| IBIS file stm32u575_585_ufqfpn48.ibs
[IBIS ver] 4.2
[File name] stm32u575_585_ufqfpn48.ibs
[File Rev] 1.0
[Date]   06-08-2021
[Source] Data Created at STMicroelectronics
[Notes]  File originated from ELDO simulations.
[Disclaimer]  This information is for modeling purpose only and is
   not guaranted. The information is subject to change without
   notice.
[Copyright] Copyright 2021 STMicroelectronics Inc.
|   Component stm32u575_585_ufqfpn48
[Component] stm32u575_585_ufqfpn48
[Manufacturer] STMicroelectronics
[Package]
| variable   typ   min   max
R_pkg   0   NA   NA
L_pkg   0   NA   NA
C_pkg   0   NA   NA
[Pin]   signal_name   model_name   R_pin   L_pin   C_pin   | Comment
1 VBAT POWER
2 PC13 io8_100m_ft_v33
3 PC14-OSC32_IN io8_100m_ft
4 PC15-OSC32_OUT io8_100m_ft
5 PH0-OSC_IN io8_100m_ft
6 PH1-OSC_OUT io8_100m_ft
7 NRST nc
8 VSSA GND
9 VDDA POWER
10 PA0 io8_100m_hslv_tamp_ft
11 PA1 io8_100m_hslv_tamp_ft
12 PA2 io8_100m_hslv_ft
13 PA3 io8_166m_hslv_ft
14 PA4 io8_100m_hslv_ft
15 PA5 io8_100m_ft
16 PA6 io8_100m_hslv_ft
17 PA7 io8_100m_hslv_ft
18 PB0 io8_100m_hslv_ft
19 PB1 io8_100m_hslv_ft
20 PB2 io8_100m_hslv_tamp_ft
21 PB10 io8_166m_hslv_i2c_ft
22 VCAP POWER
23 VSS GND
24 VDD POWER
25 PB12 io8_166m_hslv_ft
26 PB13 io8_100m_i2c_ft
27 PB14 io8_100m_i2c_ft
28 PB15 nc
29 PA8 io8_166m_hslv_ft
30 PA9 io8_100m_usb_vbus_ft
31 PA10 io8_100m_usb_id
32 PA11 io8_usb_ft
33 PA12 io8_usb_ft
34 PA13 io8_100m_ft
35 VSS GND
36 VDD POWER
37 PA14 io8_100m_ft
38 PA15 nc
39 PB3 io8_100m_i2c_ft
40 PB4 io8_100m_i2c_ft
41 PB5 io8_166m_hslv_ft
42 PB6 io8_100m_i2c_ft
43 PB7 io8_166m_hslv_i2c_ft
44 PH3-BOOT0 io8_100m_ft
45 PB8 io8_100m_i2c_ft
46 PB9 io8_100m_i2c_ft
47 VSS GND
48 VDD POWER
[Model Selector] io8_100m_ft
io8_100m_ft_hs_1v2  "IO8_FT 100MHz high speed @ 1.2V"
io8_100m_ft_hs_pu_1v2  "IO8_FT 100MHz high speed @ 1.2V pullup"
io8_100m_ft_hs_pd_1v2  "IO8_FT 100MHz high speed @ 1.2V pulldown"
io8_100m_ft_fs_1v2  "IO8_FT 100MHz fast speed @ 1.2V"
io8_100m_ft_fs_pu_1v2  "IO8_FT 100MHz fast speed @ 1.2V pullup"
io8_100m_ft_fs_pd_1v2  "IO8_FT 100MHz fast speed @ 1.2V pulldown"
io8_100m_ft_ms_1v2  "IO8_FT 100MHz med speed @ 1.2V"
io8_100m_ft_ms_pu_1v2  "IO8_FT 100MHz med speed @ 1.2V pullup"
io8_100m_ft_ms_pd_1v2  "IO8_FT 100MHz med speed @ 1.2V pulldown"
io8_100m_ft_ls_1v2  "IO8_FT 100MHz low speed @ 1.2V"
io8_100m_ft_ls_pu_1v2  "IO8_FT 100MHz low speed @ 1.2V pullup"
io8_100m_ft_ls_pd_1v2  "IO8_FT 100MHz low speed @ 1.2V pulldown"
io8_100m_ft_hs_1v8  "IO8_FT 100MHz high speed @ 1.8V"
io8_100m_ft_hs_pu_1v8  "IO8_FT 100MHz high speed @ 1.8V pullup"
io8_100m_ft_hs_pd_1v8  "IO8_FT 100MHz high speed @ 1.8V pulldown"
io8_100m_ft_fs_1v8  "IO8_FT 100MHz fast speed @ 1.8V"
io8_100m_ft_fs_pu_1v8  "IO8_FT 100MHz fast speed @ 1.8V pullup"
io8_100m_ft_fs_pd_1v8  "IO8_FT 100MHz fast speed @ 1.8V pulldown"
io8_100m_ft_ms_1v8  "IO8_FT 100MHz med speed @ 1.8V"
io8_100m_ft_ms_pu_1v8  "IO8_FT 100MHz med speed @ 1.8V pullup"
io8_100m_ft_ms_pd_1v8  "IO8_FT 100MHz med speed @ 1.8V pulldown"
io8_100m_ft_ls_1v8  "IO8_FT 100MHz low speed @ 1.8V"
io8_100m_ft_ls_pu_1v8  "IO8_FT 100MHz low speed @ 1.8V pullup"
io8_100m_ft_ls_pd_1v8  "IO8_FT 100MHz low speed @ 1.8V pulldown"
io8_100m_ft_hs_3v3  "IO8_FT 100MHz high speed @ 3.3V"
io8_100m_ft_hs_pu_3v3  "IO8_FT 100MHz high speed @ 3.3V pullup"
io8_100m_ft_hs_pd_3v3  "IO8_FT 100MHz high speed @ 3.3V pulldown"
io8_100m_ft_fs_3v3  "IO8_FT 100MHz fast speed @ 3.3V"
io8_100m_ft_fs_pu_3v3  "IO8_FT 100MHz fast speed @ 3.3V pullup"
io8_100m_ft_fs_pd_3v3  "IO8_FT 100MHz fast speed @ 3.3V pulldown"
io8_100m_ft_ms_3v3  "IO8_FT 100MHz med speed @ 3.3V"
io8_100m_ft_ms_pu_3v3  "IO8_FT 100MHz med speed @ 3.3V pullup"
io8_100m_ft_ms_pd_3v3  "IO8_FT 100MHz med speed @ 3.3V pulldown"
io8_100m_ft_ls_3v3  "IO8_FT 100MHz low speed @ 3.3V"
io8_100m_ft_ls_pu_3v3  "IO8_FT 100MHz low speed @ 3.3V pullup"
io8_100m_ft_ls_pd_3v3  "IO8_FT 100MHz low speed @ 3.3V pulldown"
[Model Selector] io8_100m_hslv_ft
io8_100m_ft_hs_1v2  "IO8_FT 100MHz high speed @ 1.2V"
io8_100m_ft_hs_pu_1v2  "IO8_FT 100MHz high speed @ 1.2V pullup"
io8_100m_ft_hs_pd_1v2  "IO8_FT 100MHz high speed @ 1.2V pulldown"
io8_100m_ft_fs_1v2  "IO8_FT 100MHz fast speed @ 1.2V"
io8_100m_ft_fs_pu_1v2  "IO8_FT 100MHz fast speed @ 1.2V pullup"
io8_100m_ft_fs_pd_1v2  "IO8_FT 100MHz fast speed @ 1.2V pulldown"
io8_100m_ft_ms_1v2  "IO8_FT 100MHz med speed @ 1.2V"
io8_100m_ft_ms_pu_1v2  "IO8_FT 100MHz med speed @ 1.2V pullup"
io8_100m_ft_ms_pd_1v2  "IO8_FT 100MHz med speed @ 1.2V pulldown"
io8_100m_ft_ls_1v2  "IO8_FT 100MHz low speed @ 1.2V"
io8_100m_ft_ls_pu_1v2  "IO8_FT 100MHz low speed @ 1.2V pullup"
io8_100m_ft_ls_pd_1v2  "IO8_FT 100MHz low speed @ 1.2V pulldown"
io8_100m_ft_hs_1v8  "IO8_FT 100MHz high speed @ 1.8V"
io8_100m_ft_hs_pu_1v8  "IO8_FT 100MHz high speed @ 1.8V pullup"
io8_100m_ft_hs_pd_1v8  "IO8_FT 100MHz high speed @ 1.8V pulldown"
io8_100m_ft_fs_1v8  "IO8_FT 100MHz fast speed @ 1.8V"
io8_100m_ft_fs_pu_1v8  "IO8_FT 100MHz fast speed @ 1.8V pullup"
io8_100m_ft_fs_pd_1v8  "IO8_FT 100MHz fast speed @ 1.8V pulldown"
io8_100m_ft_ms_1v8  "IO8_FT 100MHz med speed @ 1.8V"
io8_100m_ft_ms_pu_1v8  "IO8_FT 100MHz med speed @ 1.8V pullup"
io8_100m_ft_ms_pd_1v8  "IO8_FT 100MHz med speed @ 1.8V pulldown"
io8_100m_ft_ls_1v8  "IO8_FT 100MHz low speed @ 1.8V"
io8_100m_ft_ls_pu_1v8  "IO8_FT 100MHz low speed @ 1.8V pullup"
io8_100m_ft_ls_pd_1v8  "IO8_FT 100MHz low speed @ 1.8V pulldown"
io8_100m_ft_hs_3v3  "IO8_FT 100MHz high speed @ 3.3V"
io8_100m_ft_hs_pu_3v3  "IO8_FT 100MHz high speed @ 3.3V pullup"
io8_100m_ft_hs_pd_3v3  "IO8_FT 100MHz high speed @ 3.3V pulldown"
io8_100m_ft_fs_3v3  "IO8_FT 100MHz fast speed @ 3.3V"
io8_100m_ft_fs_pu_3v3  "IO8_FT 100MHz fast speed @ 3.3V pullup"
io8_100m_ft_fs_pd_3v3  "IO8_FT 100MHz fast speed @ 3.3V pulldown"
io8_100m_ft_ms_3v3  "IO8_FT 100MHz med speed @ 3.3V"
io8_100m_ft_ms_pu_3v3  "IO8_FT 100MHz med speed @ 3.3V pullup"
io8_100m_ft_ms_pd_3v3  "IO8_FT 100MHz med speed @ 3.3V pulldown"
io8_100m_ft_ls_3v3  "IO8_FT 100MHz low speed @ 3.3V"
io8_100m_ft_ls_pu_3v3  "IO8_FT 100MHz low speed @ 3.3V pullup"
io8_100m_ft_ls_pd_3v3  "IO8_FT 100MHz low speed @ 3.3V pulldown"
io8_100m_hslv_ft_hs_1v2  "IO8_FT 100MHz HSLV high speed @ 1.2V"
io8_100m_hslv_ft_hs_pu_1v2  "IO8_FT 100MHz HSLV high speed @ 1.2V pullup"
io8_100m_hslv_ft_hs_pd_1v2  "IO8_FT 100MHz HSLV high speed @ 1.2V pulldown"
io8_100m_hslv_ft_fs_1v2  "IO8_FT 100MHz HSLV fast speed @ 1.2V"
io8_100m_hslv_ft_fs_pu_1v2  "IO8_FT 100MHz HSLV fast speed @ 1.2V pullup"
io8_100m_hslv_ft_fs_pd_1v2  "IO8_FT 100MHz HSLV fast speed @ 1.2V pulldown"
io8_100m_hslv_ft_ms_1v2  "IO8_FT 100MHz HSLV med speed @ 1.2V"
io8_100m_hslv_ft_ms_pu_1v2  "IO8_FT 100MHz HSLV med speed @ 1.2V pullup"
io8_100m_hslv_ft_ms_pd_1v2  "IO8_FT 100MHz HSLV med speed @ 1.2V pulldown"
io8_100m_hslv_ft_ls_1v2  "IO8_FT 100MHz HSLV low speed @ 1.2V"
io8_100m_hslv_ft_ls_pu_1v2  "IO8_FT 100MHz HSLV low speed @ 1.2V pullup"
io8_100m_hslv_ft_ls_pd_1v2  "IO8_FT 100MHz HSLV low speed @ 1.2V pulldown"
io8_100m_hslv_ft_hs_1v8  "IO8_FT 100MHz HSLV high speed @ 1.8V"
io8_100m_hslv_ft_hs_pu_1v8  "IO8_FT 100MHz HSLV high speed @ 1.8V pullup"
io8_100m_hslv_ft_hs_pd_1v8  "IO8_FT 100MHz HSLV high speed @ 1.8V pulldown"
io8_100m_hslv_ft_fs_1v8  "IO8_FT 100MHz HSLV fast speed @ 1.8V"
io8_100m_hslv_ft_fs_pu_1v8  "IO8_FT 100MHz HSLV fast speed @ 1.8V pullup"
io8_100m_hslv_ft_fs_pd_1v8  "IO8_FT 100MHz HSLV fast speed @ 1.8V pulldown"
io8_100m_hslv_ft_ms_1v8  "IO8_FT 100MHz HSLV med speed @ 1.8V"
io8_100m_hslv_ft_ms_pu_1v8  "IO8_FT 100MHz HSLV med speed @ 1.8V pullup"
io8_100m_hslv_ft_ms_pd_1v8  "IO8_FT 100MHz HSLV med speed @ 1.8V pulldown"
io8_100m_hslv_ft_ls_1v8  "IO8_FT 100MHz HSLV low speed @ 1.8V"
io8_100m_hslv_ft_ls_pu_1v8  "IO8_FT 100MHz HSLV low speed @ 1.8V pullup"
io8_100m_hslv_ft_ls_pd_1v8  "IO8_FT 100MHz HSLV low speed @ 1.8V pulldown"
io8_100m_hslv_ft_hs_2v5  "IO8_FT 100MHz HSLV high speed @ 2.5V"
io8_100m_hslv_ft_hs_pu_2v5  "IO8_FT 100MHz HSLV high speed @ 2.5V pullup"
io8_100m_hslv_ft_hs_pd_2v5  "IO8_FT 100MHz HSLV high speed @ 2.5V pulldown"
io8_100m_hslv_ft_fs_2v5  "IO8_FT 100MHz HSLV fast speed @ 2.5V"
io8_100m_hslv_ft_fs_pu_2v5  "IO8_FT 100MHz HSLV fast speed @ 2.5V pullup"
io8_100m_hslv_ft_fs_pd_2v5  "IO8_FT 100MHz HSLV fast speed @ 2.5V pulldown"
io8_100m_hslv_ft_ms_2v5  "IO8_FT 100MHz HSLV med speed @ 2.5V"
io8_100m_hslv_ft_ms_pu_2v5  "IO8_FT 100MHz HSLV med speed @ 2.5V pullup"
io8_100m_hslv_ft_ms_pd_2v5  "IO8_FT 100MHz HSLV med speed @ 2.5V pulldown"
io8_100m_hslv_ft_ls_2v5  "IO8_FT 100MHz HSLV low speed @ 2.5V"
io8_100m_hslv_ft_ls_pu_2v5  "IO8_FT 100MHz HSLV low speed @ 2.5V pullup"
io8_100m_hslv_ft_ls_pd_2v5  "IO8_FT 100MHz HSLV low speed @ 2.5V pulldown"
[Model Selector] io8_166m_hslv_ft
io8_166m_ft_hs_1v2  "IO8_FT 166MHz high speed @ 1.2V"
io8_166m_ft_hs_pu_1v2  "IO8_FT 166MHz high speed @ 1.2V pullup"
io8_166m_ft_hs_pd_1v2  "IO8_FT 166MHz high speed @ 1.2V pulldown"
io8_166m_ft_fs_1v2  "IO8_FT 166MHz fast speed @ 1.2V"
io8_166m_ft_fs_pu_1v2  "IO8_FT 166MHz fast speed @ 1.2V pullup"
io8_166m_ft_fs_pd_1v2  "IO8_FT 166MHz fast speed @ 1.2V pulldown"
io8_166m_ft_ms_1v2  "IO8_FT 166MHz med speed @ 1.2V"
io8_166m_ft_ms_pu_1v2  "IO8_FT 166MHz med speed @ 1.2V pullup"
io8_166m_ft_ms_pd_1v2  "IO8_FT 166MHz med speed @ 1.2V pulldown"
io8_166m_ft_ls_1v2  "IO8_FT 166MHz low speed @ 1.2V"
io8_166m_ft_ls_pu_1v2  "IO8_FT 166MHz low speed @ 1.2V pullup"
io8_166m_ft_ls_pd_1v2  "IO8_FT 166MHz low speed @ 1.2V pulldown"
io8_166m_ft_hs_1v8  "IO8_FT 166MHz high speed @ 1.8V"
io8_166m_ft_hs_pu_1v8  "IO8_FT 166MHz high speed @ 1.8V pullup"
io8_166m_ft_hs_pd_1v8  "IO8_FT 166MHz high speed @ 1.8V pulldown"
io8_166m_ft_fs_1v8  "IO8_FT 166MHz fast speed @ 1.8V"
io8_166m_ft_fs_pu_1v8  "IO8_FT 166MHz fast speed @ 1.8V pullup"
io8_166m_ft_fs_pd_1v8  "IO8_FT 166MHz fast speed @ 1.8V pulldown"
io8_166m_ft_ms_1v8  "IO8_FT 166MHz med speed @ 1.8V"
io8_166m_ft_ms_pu_1v8  "IO8_FT 166MHz med speed @ 1.8V pullup"
io8_166m_ft_ms_pd_1v8  "IO8_FT 166MHz med speed @ 1.8V pulldown"
io8_166m_ft_ls_1v8  "IO8_FT 166MHz low speed @ 1.8V"
io8_166m_ft_ls_pu_1v8  "IO8_FT 166MHz low speed @ 1.8V pullup"
io8_166m_ft_ls_pd_1v8  "IO8_FT 166MHz low speed @ 1.8V pulldown"
io8_166m_ft_hs_3v3  "IO8_FT 166MHz high speed @ 3.3V"
io8_166m_ft_hs_pu_3v3  "IO8_FT 166MHz high speed @ 3.3V pullup"
io8_166m_ft_hs_pd_3v3  "IO8_FT 166MHz high speed @ 3.3V pulldown"
io8_166m_ft_fs_3v3  "IO8_FT 166MHz fast speed @ 3.3V"
io8_166m_ft_fs_pu_3v3  "IO8_FT 166MHz fast speed @ 3.3V pullup"
io8_166m_ft_fs_pd_3v3  "IO8_FT 166MHz fast speed @ 3.3V pulldown"
io8_166m_ft_ms_3v3  "IO8_FT 166MHz med speed @ 3.3V"
io8_166m_ft_ms_pu_3v3  "IO8_FT 166MHz med speed @ 3.3V pullup"
io8_166m_ft_ms_pd_3v3  "IO8_FT 166MHz med speed @ 3.3V pulldown"
io8_166m_ft_ls_3v3  "IO8_FT 166MHz low speed @ 3.3V"
io8_166m_ft_ls_pu_3v3  "IO8_FT 166MHz low speed @ 3.3V pullup"
io8_166m_ft_ls_pd_3v3  "IO8_FT 166MHz low speed @ 3.3V pulldown"
io8_166m_hslv_ft_hs_1v2  "IO8_FT 166MHz HSLV high speed @ 1.2V"
io8_166m_hslv_ft_hs_pu_1v2  "IO8_FT 166MHz HSLV high speed @ 1.2V pullup"
io8_166m_hslv_ft_hs_pd_1v2  "IO8_FT 166MHz HSLV high speed @ 1.2V pulldown"
io8_166m_hslv_ft_fs_1v2  "IO8_FT 166MHz HSLV fast speed @ 1.2V"
io8_166m_hslv_ft_fs_pu_1v2  "IO8_FT 166MHz HSLV fast speed @ 1.2V pullup"
io8_166m_hslv_ft_fs_pd_1v2  "IO8_FT 166MHz HSLV fast speed @ 1.2V pulldown"
io8_166m_hslv_ft_ms_1v2  "IO8_FT 166MHz HSLV med speed @ 1.2V"
io8_166m_hslv_ft_ms_pu_1v2  "IO8_FT 166MHz HSLV med speed @ 1.2V pullup"
io8_166m_hslv_ft_ms_pd_1v2  "IO8_FT 166MHz HSLV med speed @ 1.2V pulldown"
io8_166m_hslv_ft_ls_1v2  "IO8_FT 166MHz HSLV low speed @ 1.2V"
io8_166m_hslv_ft_ls_pu_1v2  "IO8_FT 166MHz HSLV low speed @ 1.2V pullup"
io8_166m_hslv_ft_ls_pd_1v2  "IO8_FT 166MHz HSLV low speed @ 1.2V pulldown"
io8_166m_hslv_ft_hs_1v8  "IO8_FT 166MHz HSLV high speed @ 1.8V"
io8_166m_hslv_ft_hs_pu_1v8  "IO8_FT 166MHz HSLV high speed @ 1.8V pullup"
io8_166m_hslv_ft_hs_pd_1v8  "IO8_FT 166MHz HSLV high speed @ 1.8V pulldown"
io8_166m_hslv_ft_fs_1v8  "IO8_FT 166MHz HSLV fast speed @ 1.8V"
io8_166m_hslv_ft_fs_pu_1v8  "IO8_FT 166MHz HSLV fast speed @ 1.8V pullup"
io8_166m_hslv_ft_fs_pd_1v8  "IO8_FT 166MHz HSLV fast speed @ 1.8V pulldown"
io8_166m_hslv_ft_ms_1v8  "IO8_FT 166MHz HSLV med speed @ 1.8V"
io8_166m_hslv_ft_ms_pu_1v8  "IO8_FT 166MHz HSLV med speed @ 1.8V pullup"
io8_166m_hslv_ft_ms_pd_1v8  "IO8_FT 166MHz HSLV med speed @ 1.8V pulldown"
io8_166m_hslv_ft_ls_1v8  "IO8_FT 166MHz HSLV low speed @ 1.8V"
io8_166m_hslv_ft_ls_pu_1v8  "IO8_FT 166MHz HSLV low speed @ 1.8V pullup"
io8_166m_hslv_ft_ls_pd_1v8  "IO8_FT 166MHz HSLV low speed @ 1.8V pulldown"
io8_166m_hslv_ft_hs_2v5  "IO8_FT 166MHz HSLV high speed @ 2.5V"
io8_166m_hslv_ft_hs_pu_2v5  "IO8_FT 166MHz HSLV high speed @ 2.5V pullup"
io8_166m_hslv_ft_hs_pd_2v5  "IO8_FT 166MHz HSLV high speed @ 2.5V pulldown"
io8_166m_hslv_ft_fs_2v5  "IO8_FT 166MHz HSLV fast speed @ 2.5V"
io8_166m_hslv_ft_fs_pu_2v5  "IO8_FT 166MHz HSLV fast speed @ 2.5V pullup"
io8_166m_hslv_ft_fs_pd_2v5  "IO8_FT 166MHz HSLV fast speed @ 2.5V pulldown"
io8_166m_hslv_ft_ms_2v5  "IO8_FT 166MHz HSLV med speed @ 2.5V"
io8_166m_hslv_ft_ms_pu_2v5  "IO8_FT 166MHz HSLV med speed @ 2.5V pullup"
io8_166m_hslv_ft_ms_pd_2v5  "IO8_FT 166MHz HSLV med speed @ 2.5V pulldown"
io8_166m_hslv_ft_ls_2v5  "IO8_FT 166MHz HSLV low speed @ 2.5V"
io8_166m_hslv_ft_ls_pu_2v5  "IO8_FT 166MHz HSLV low speed @ 2.5V pullup"
io8_166m_hslv_ft_ls_pd_2v5  "IO8_FT 166MHz HSLV low speed @ 2.5V pulldown"
[Model Selector] io8_100m_ft_v33
io8_ft_v33_hs_1v2  "IO8_FT_V33 high speed @ 1.2V"
io8_ft_v33_hs_pu_1v2  "IO8_FT_V33 high speed @ 1.2V pullup"
io8_ft_v33_hs_pd_1v2  "IO8_FT_V33 high speed @ 1.2V pulldown"
io8_ft_v33_fs_1v2  "IO8_FT_V33 fast speed @ 1.2V"
io8_ft_v33_fs_pu_1v2  "IO8_FT_V33 fast speed @ 1.2V pullup"
io8_ft_v33_fs_pd_1v2  "IO8_FT_V33 fast speed @ 1.2V pulldown"
io8_ft_v33_ms_1v2  "IO8_FT_V33 med speed @ 1.2V"
io8_ft_v33_ms_pu_1v2  "IO8_FT_V33 med speed @ 1.2V pullup"
io8_ft_v33_ms_pd_1v2  "IO8_FT_V33 med speed @ 1.2V pulldown"
io8_ft_v33_ls_1v2  "IO8_FT_V33 low speed @ 1.2V"
io8_ft_v33_ls_pu_1v2  "IO8_FT_V33 low speed @ 1.2V pullup"
io8_ft_v33_ls_pd_1v2  "IO8_FT_V33 low speed @ 1.2V pulldown"
io8_ft_v33_hs_1v8  "IO8_FT_V33 high speed @ 1.8V"
io8_ft_v33_hs_pu_1v8  "IO8_FT_V33 high speed @ 1.8V pullup"
io8_ft_v33_hs_pd_1v8  "IO8_FT_V33 high speed @ 1.8V pulldown"
io8_ft_v33_fs_1v8  "IO8_FT_V33 fast speed @ 1.8V"
io8_ft_v33_fs_pu_1v8  "IO8_FT_V33 fast speed @ 1.8V pullup"
io8_ft_v33_fs_pd_1v8  "IO8_FT_V33 fast speed @ 1.8V pulldown"
io8_ft_v33_ms_1v8  "IO8_FT_V33 med speed @ 1.8V"
io8_ft_v33_ms_pu_1v8  "IO8_FT_V33 med speed @ 1.8V pullup"
io8_ft_v33_ms_pd_1v8  "IO8_FT_V33 med speed @ 1.8V pulldown"
io8_ft_v33_ls_1v8  "IO8_FT_V33 low speed @ 1.8V"
io8_ft_v33_ls_pu_1v8  "IO8_FT_V33 low speed @ 1.8V pullup"
io8_ft_v33_ls_pd_1v8  "IO8_FT_V33 low speed @ 1.8V pulldown"
io8_ft_v33_hs_3v3  "IO8_FT_V33 high speed @ 3.3V"
io8_ft_v33_hs_pu_3v3  "IO8_FT_V33 high speed @ 3.3V pullup"
io8_ft_v33_hs_pd_3v3  "IO8_FT_V33 high speed @ 3.3V pulldown"
io8_ft_v33_fs_3v3  "IO8_FT_V33 fast speed @ 3.3V"
io8_ft_v33_fs_pu_3v3  "IO8_FT_V33 fast speed @ 3.3V pullup"
io8_ft_v33_fs_pd_3v3  "IO8_FT_V33 fast speed @ 3.3V pulldown"
io8_ft_v33_ms_3v3  "IO8_FT_V33 med speed @ 3.3V"
io8_ft_v33_ms_pu_3v3  "IO8_FT_V33 med speed @ 3.3V pullup"
io8_ft_v33_ms_pd_3v3  "IO8_FT_V33 med speed @ 3.3V pulldown"
io8_ft_v33_ls_3v3  "IO8_FT_V33 low speed @ 3.3V"
io8_ft_v33_ls_pu_3v3  "IO8_FT_V33 low speed @ 3.3V pullup"
io8_ft_v33_ls_pd_3v3  "IO8_FT_V33 low speed @ 3.3V pulldown"
[Model Selector] io8_100m_hslv_tamp_ft
io8_100m_ft_hs_1v2  "IO8_FT 100MHz high speed @ 1.2V"
io8_100m_ft_hs_pu_1v2  "IO8_FT 100MHz high speed @ 1.2V pullup"
io8_100m_ft_hs_pd_1v2  "IO8_FT 100MHz high speed @ 1.2V pulldown"
io8_100m_ft_fs_1v2  "IO8_FT 100MHz fast speed @ 1.2V"
io8_100m_ft_fs_pu_1v2  "IO8_FT 100MHz fast speed @ 1.2V pullup"
io8_100m_ft_fs_pd_1v2  "IO8_FT 100MHz fast speed @ 1.2V pulldown"
io8_100m_ft_ms_1v2  "IO8_FT 100MHz med speed @ 1.2V"
io8_100m_ft_ms_pu_1v2  "IO8_FT 100MHz med speed @ 1.2V pullup"
io8_100m_ft_ms_pd_1v2  "IO8_FT 100MHz med speed @ 1.2V pulldown"
io8_100m_ft_ls_1v2  "IO8_FT 100MHz low speed @ 1.2V"
io8_100m_ft_ls_pu_1v2  "IO8_FT 100MHz low speed @ 1.2V pullup"
io8_100m_ft_ls_pd_1v2  "IO8_FT 100MHz low speed @ 1.2V pulldown"
io8_100m_ft_hs_1v8  "IO8_FT 100MHz high speed @ 1.8V"
io8_100m_ft_hs_pu_1v8  "IO8_FT 100MHz high speed @ 1.8V pullup"
io8_100m_ft_hs_pd_1v8  "IO8_FT 100MHz high speed @ 1.8V pulldown"
io8_100m_ft_fs_1v8  "IO8_FT 100MHz fast speed @ 1.8V"
io8_100m_ft_fs_pu_1v8  "IO8_FT 100MHz fast speed @ 1.8V pullup"
io8_100m_ft_fs_pd_1v8  "IO8_FT 100MHz fast speed @ 1.8V pulldown"
io8_100m_ft_ms_1v8  "IO8_FT 100MHz med speed @ 1.8V"
io8_100m_ft_ms_pu_1v8  "IO8_FT 100MHz med speed @ 1.8V pullup"
io8_100m_ft_ms_pd_1v8  "IO8_FT 100MHz med speed @ 1.8V pulldown"
io8_100m_ft_ls_1v8  "IO8_FT 100MHz low speed @ 1.8V"
io8_100m_ft_ls_pu_1v8  "IO8_FT 100MHz low speed @ 1.8V pullup"
io8_100m_ft_ls_pd_1v8  "IO8_FT 100MHz low speed @ 1.8V pulldown"
io8_100m_ft_hs_3v3  "IO8_FT 100MHz high speed @ 3.3V"
io8_100m_ft_hs_pu_3v3  "IO8_FT 100MHz high speed @ 3.3V pullup"
io8_100m_ft_hs_pd_3v3  "IO8_FT 100MHz high speed @ 3.3V pulldown"
io8_100m_ft_fs_3v3  "IO8_FT 100MHz fast speed @ 3.3V"
io8_100m_ft_fs_pu_3v3  "IO8_FT 100MHz fast speed @ 3.3V pullup"
io8_100m_ft_fs_pd_3v3  "IO8_FT 100MHz fast speed @ 3.3V pulldown"
io8_100m_ft_ms_3v3  "IO8_FT 100MHz med speed @ 3.3V"
io8_100m_ft_ms_pu_3v3  "IO8_FT 100MHz med speed @ 3.3V pullup"
io8_100m_ft_ms_pd_3v3  "IO8_FT 100MHz med speed @ 3.3V pulldown"
io8_100m_ft_ls_3v3  "IO8_FT 100MHz low speed @ 3.3V"
io8_100m_ft_ls_pu_3v3  "IO8_FT 100MHz low speed @ 3.3V pullup"
io8_100m_ft_ls_pd_3v3  "IO8_FT 100MHz low speed @ 3.3V pulldown"
io8_100m_hslv_ft_hs_1v2  "IO8_FT 100MHz HSLV high speed @ 1.2V"
io8_100m_hslv_ft_hs_pu_1v2  "IO8_FT 100MHz HSLV high speed @ 1.2V pullup"
io8_100m_hslv_ft_hs_pd_1v2  "IO8_FT 100MHz HSLV high speed @ 1.2V pulldown"
io8_100m_hslv_ft_fs_1v2  "IO8_FT 100MHz HSLV fast speed @ 1.2V"
io8_100m_hslv_ft_fs_pu_1v2  "IO8_FT 100MHz HSLV fast speed @ 1.2V pullup"
io8_100m_hslv_ft_fs_pd_1v2  "IO8_FT 100MHz HSLV fast speed @ 1.2V pulldown"
io8_100m_hslv_ft_ms_1v2  "IO8_FT 100MHz HSLV med speed @ 1.2V"
io8_100m_hslv_ft_ms_pu_1v2  "IO8_FT 100MHz HSLV med speed @ 1.2V pullup"
io8_100m_hslv_ft_ms_pd_1v2  "IO8_FT 100MHz HSLV med speed @ 1.2V pulldown"
io8_100m_hslv_ft_ls_1v2  "IO8_FT 100MHz HSLV low speed @ 1.2V"
io8_100m_hslv_ft_ls_pu_1v2  "IO8_FT 100MHz HSLV low speed @ 1.2V pullup"
io8_100m_hslv_ft_ls_pd_1v2  "IO8_FT 100MHz HSLV low speed @ 1.2V pulldown"
io8_100m_hslv_ft_hs_1v8  "IO8_FT 100MHz HSLV high speed @ 1.8V"
io8_100m_hslv_ft_hs_pu_1v8  "IO8_FT 100MHz HSLV high speed @ 1.8V pullup"
io8_100m_hslv_ft_hs_pd_1v8  "IO8_FT 100MHz HSLV high speed @ 1.8V pulldown"
io8_100m_hslv_ft_fs_1v8  "IO8_FT 100MHz HSLV fast speed @ 1.8V"
io8_100m_hslv_ft_fs_pu_1v8  "IO8_FT 100MHz HSLV fast speed @ 1.8V pullup"
io8_100m_hslv_ft_fs_pd_1v8  "IO8_FT 100MHz HSLV fast speed @ 1.8V pulldown"
io8_100m_hslv_ft_ms_1v8  "IO8_FT 100MHz HSLV med speed @ 1.8V"
io8_100m_hslv_ft_ms_pu_1v8  "IO8_FT 100MHz HSLV med speed @ 1.8V pullup"
io8_100m_hslv_ft_ms_pd_1v8  "IO8_FT 100MHz HSLV med speed @ 1.8V pulldown"
io8_100m_hslv_ft_ls_1v8  "IO8_FT 100MHz HSLV low speed @ 1.8V"
io8_100m_hslv_ft_ls_pu_1v8  "IO8_FT 100MHz HSLV low speed @ 1.8V pullup"
io8_100m_hslv_ft_ls_pd_1v8  "IO8_FT 100MHz HSLV low speed @ 1.8V pulldown"
io8_100m_hslv_ft_hs_2v5  "IO8_FT 100MHz HSLV high speed @ 2.5V"
io8_100m_hslv_ft_hs_pu_2v5  "IO8_FT 100MHz HSLV high speed @ 2.5V pullup"
io8_100m_hslv_ft_hs_pd_2v5  "IO8_FT 100MHz HSLV high speed @ 2.5V pulldown"
io8_100m_hslv_ft_fs_2v5  "IO8_FT 100MHz HSLV fast speed @ 2.5V"
io8_100m_hslv_ft_fs_pu_2v5  "IO8_FT 100MHz HSLV fast speed @ 2.5V pullup"
io8_100m_hslv_ft_fs_pd_2v5  "IO8_FT 100MHz HSLV fast speed @ 2.5V pulldown"
io8_100m_hslv_ft_ms_2v5  "IO8_FT 100MHz HSLV med speed @ 2.5V"
io8_100m_hslv_ft_ms_pu_2v5  "IO8_FT 100MHz HSLV med speed @ 2.5V pullup"
io8_100m_hslv_ft_ms_pd_2v5  "IO8_FT 100MHz HSLV med speed @ 2.5V pulldown"
io8_100m_hslv_ft_ls_2v5  "IO8_FT 100MHz HSLV low speed @ 2.5V"
io8_100m_hslv_ft_ls_pu_2v5  "IO8_FT 100MHz HSLV low speed @ 2.5V pullup"
io8_100m_hslv_ft_ls_pd_2v5  "IO8_FT 100MHz HSLV low speed @ 2.5V pulldown"
io8_ft_v33_hs_1v2  "IO8_FT_V33 high speed @ 1.2V"
io8_ft_v33_hs_pu_1v2  "IO8_FT_V33 high speed @ 1.2V pullup"
io8_ft_v33_hs_pd_1v2  "IO8_FT_V33 high speed @ 1.2V pulldown"
io8_ft_v33_fs_1v2  "IO8_FT_V33 fast speed @ 1.2V"
io8_ft_v33_fs_pu_1v2  "IO8_FT_V33 fast speed @ 1.2V pullup"
io8_ft_v33_fs_pd_1v2  "IO8_FT_V33 fast speed @ 1.2V pulldown"
io8_ft_v33_ms_1v2  "IO8_FT_V33 med speed @ 1.2V"
io8_ft_v33_ms_pu_1v2  "IO8_FT_V33 med speed @ 1.2V pullup"
io8_ft_v33_ms_pd_1v2  "IO8_FT_V33 med speed @ 1.2V pulldown"
io8_ft_v33_ls_1v2  "IO8_FT_V33 low speed @ 1.2V"
io8_ft_v33_ls_pu_1v2  "IO8_FT_V33 low speed @ 1.2V pullup"
io8_ft_v33_ls_pd_1v2  "IO8_FT_V33 low speed @ 1.2V pulldown"
io8_ft_v33_hs_1v8  "IO8_FT_V33 high speed @ 1.8V"
io8_ft_v33_hs_pu_1v8  "IO8_FT_V33 high speed @ 1.8V pullup"
io8_ft_v33_hs_pd_1v8  "IO8_FT_V33 high speed @ 1.8V pulldown"
io8_ft_v33_fs_1v8  "IO8_FT_V33 fast speed @ 1.8V"
io8_ft_v33_fs_pu_1v8  "IO8_FT_V33 fast speed @ 1.8V pullup"
io8_ft_v33_fs_pd_1v8  "IO8_FT_V33 fast speed @ 1.8V pulldown"
io8_ft_v33_ms_1v8  "IO8_FT_V33 med speed @ 1.8V"
io8_ft_v33_ms_pu_1v8  "IO8_FT_V33 med speed @ 1.8V pullup"
io8_ft_v33_ms_pd_1v8  "IO8_FT_V33 med speed @ 1.8V pulldown"
io8_ft_v33_ls_1v8  "IO8_FT_V33 low speed @ 1.8V"
io8_ft_v33_ls_pu_1v8  "IO8_FT_V33 low speed @ 1.8V pullup"
io8_ft_v33_ls_pd_1v8  "IO8_FT_V33 low speed @ 1.8V pulldown"
io8_ft_v33_hs_3v3  "IO8_FT_V33 high speed @ 3.3V"
io8_ft_v33_hs_pu_3v3  "IO8_FT_V33 high speed @ 3.3V pullup"
io8_ft_v33_hs_pd_3v3  "IO8_FT_V33 high speed @ 3.3V pulldown"
io8_ft_v33_fs_3v3  "IO8_FT_V33 fast speed @ 3.3V"
io8_ft_v33_fs_pu_3v3  "IO8_FT_V33 fast speed @ 3.3V pullup"
io8_ft_v33_fs_pd_3v3  "IO8_FT_V33 fast speed @ 3.3V pulldown"
io8_ft_v33_ms_3v3  "IO8_FT_V33 med speed @ 3.3V"
io8_ft_v33_ms_pu_3v3  "IO8_FT_V33 med speed @ 3.3V pullup"
io8_ft_v33_ms_pd_3v3  "IO8_FT_V33 med speed @ 3.3V pulldown"
io8_ft_v33_ls_3v3  "IO8_FT_V33 low speed @ 3.3V"
io8_ft_v33_ls_pu_3v3  "IO8_FT_V33 low speed @ 3.3V pullup"
io8_ft_v33_ls_pd_3v3  "IO8_FT_V33 low speed @ 3.3V pulldown"
[Model Selector] io8_100m_usb_id
io8_100m_ft_hs_1v2  "IO8_FT 100MHz high speed @ 1.2V"
io8_100m_ft_hs_pu_1v2  "IO8_FT 100MHz high speed @ 1.2V pullup"
io8_100m_ft_hs_pd_1v2  "IO8_FT 100MHz high speed @ 1.2V pulldown"
io8_100m_ft_fs_1v2  "IO8_FT 100MHz fast speed @ 1.2V"
io8_100m_ft_fs_pu_1v2  "IO8_FT 100MHz fast speed @ 1.2V pullup"
io8_100m_ft_fs_pd_1v2  "IO8_FT 100MHz fast speed @ 1.2V pulldown"
io8_100m_ft_ms_1v2  "IO8_FT 100MHz med speed @ 1.2V"
io8_100m_ft_ms_pu_1v2  "IO8_FT 100MHz med speed @ 1.2V pullup"
io8_100m_ft_ms_pd_1v2  "IO8_FT 100MHz med speed @ 1.2V pulldown"
io8_100m_ft_ls_1v2  "IO8_FT 100MHz low speed @ 1.2V"
io8_100m_ft_ls_pu_1v2  "IO8_FT 100MHz low speed @ 1.2V pullup"
io8_100m_ft_ls_pd_1v2  "IO8_FT 100MHz low speed @ 1.2V pulldown"
io8_100m_ft_hs_1v8  "IO8_FT 100MHz high speed @ 1.8V"
io8_100m_ft_hs_pu_1v8  "IO8_FT 100MHz high speed @ 1.8V pullup"
io8_100m_ft_hs_pd_1v8  "IO8_FT 100MHz high speed @ 1.8V pulldown"
io8_100m_ft_fs_1v8  "IO8_FT 100MHz fast speed @ 1.8V"
io8_100m_ft_fs_pu_1v8  "IO8_FT 100MHz fast speed @ 1.8V pullup"
io8_100m_ft_fs_pd_1v8  "IO8_FT 100MHz fast speed @ 1.8V pulldown"
io8_100m_ft_ms_1v8  "IO8_FT 100MHz med speed @ 1.8V"
io8_100m_ft_ms_pu_1v8  "IO8_FT 100MHz med speed @ 1.8V pullup"
io8_100m_ft_ms_pd_1v8  "IO8_FT 100MHz med speed @ 1.8V pulldown"
io8_100m_ft_ls_1v8  "IO8_FT 100MHz low speed @ 1.8V"
io8_100m_ft_ls_pu_1v8  "IO8_FT 100MHz low speed @ 1.8V pullup"
io8_100m_ft_ls_pd_1v8  "IO8_FT 100MHz low speed @ 1.8V pulldown"
io8_100m_ft_hs_3v3  "IO8_FT 100MHz high speed @ 3.3V"
io8_100m_ft_hs_pu_3v3  "IO8_FT 100MHz high speed @ 3.3V pullup"
io8_100m_ft_hs_pd_3v3  "IO8_FT 100MHz high speed @ 3.3V pulldown"
io8_100m_ft_fs_3v3  "IO8_FT 100MHz fast speed @ 3.3V"
io8_100m_ft_fs_pu_3v3  "IO8_FT 100MHz fast speed @ 3.3V pullup"
io8_100m_ft_fs_pd_3v3  "IO8_FT 100MHz fast speed @ 3.3V pulldown"
io8_100m_ft_ms_3v3  "IO8_FT 100MHz med speed @ 3.3V"
io8_100m_ft_ms_pu_3v3  "IO8_FT 100MHz med speed @ 3.3V pullup"
io8_100m_ft_ms_pd_3v3  "IO8_FT 100MHz med speed @ 3.3V pulldown"
io8_100m_ft_ls_3v3  "IO8_FT 100MHz low speed @ 3.3V"
io8_100m_ft_ls_pu_3v3  "IO8_FT 100MHz low speed @ 3.3V pullup"
io8_100m_ft_ls_pd_3v3  "IO8_FT 100MHz low speed @ 3.3V pulldown"
io8usb_id_nopu  "IOUSB ID @ 3.3V"
io8usb_id_pu  "IOUSB ID @ 3.3V pullup"
[Model Selector] io8_100m_usb_vbus_ft
io8_100m_ft_hs_1v2  "IO8_FT 100MHz high speed @ 1.2V"
io8_100m_ft_hs_pu_1v2  "IO8_FT 100MHz high speed @ 1.2V pullup"
io8_100m_ft_hs_pd_1v2  "IO8_FT 100MHz high speed @ 1.2V pulldown"
io8_100m_ft_fs_1v2  "IO8_FT 100MHz fast speed @ 1.2V"
io8_100m_ft_fs_pu_1v2  "IO8_FT 100MHz fast speed @ 1.2V pullup"
io8_100m_ft_fs_pd_1v2  "IO8_FT 100MHz fast speed @ 1.2V pulldown"
io8_100m_ft_ms_1v2  "IO8_FT 100MHz med speed @ 1.2V"
io8_100m_ft_ms_pu_1v2  "IO8_FT 100MHz med speed @ 1.2V pullup"
io8_100m_ft_ms_pd_1v2  "IO8_FT 100MHz med speed @ 1.2V pulldown"
io8_100m_ft_ls_1v2  "IO8_FT 100MHz low speed @ 1.2V"
io8_100m_ft_ls_pu_1v2  "IO8_FT 100MHz low speed @ 1.2V pullup"
io8_100m_ft_ls_pd_1v2  "IO8_FT 100MHz low speed @ 1.2V pulldown"
io8_100m_ft_hs_1v8  "IO8_FT 100MHz high speed @ 1.8V"
io8_100m_ft_hs_pu_1v8  "IO8_FT 100MHz high speed @ 1.8V pullup"
io8_100m_ft_hs_pd_1v8  "IO8_FT 100MHz high speed @ 1.8V pulldown"
io8_100m_ft_fs_1v8  "IO8_FT 100MHz fast speed @ 1.8V"
io8_100m_ft_fs_pu_1v8  "IO8_FT 100MHz fast speed @ 1.8V pullup"
io8_100m_ft_fs_pd_1v8  "IO8_FT 100MHz fast speed @ 1.8V pulldown"
io8_100m_ft_ms_1v8  "IO8_FT 100MHz med speed @ 1.8V"
io8_100m_ft_ms_pu_1v8  "IO8_FT 100MHz med speed @ 1.8V pullup"
io8_100m_ft_ms_pd_1v8  "IO8_FT 100MHz med speed @ 1.8V pulldown"
io8_100m_ft_ls_1v8  "IO8_FT 100MHz low speed @ 1.8V"
io8_100m_ft_ls_pu_1v8  "IO8_FT 100MHz low speed @ 1.8V pullup"
io8_100m_ft_ls_pd_1v8  "IO8_FT 100MHz low speed @ 1.8V pulldown"
io8_100m_ft_hs_3v3  "IO8_FT 100MHz high speed @ 3.3V"
io8_100m_ft_hs_pu_3v3  "IO8_FT 100MHz high speed @ 3.3V pullup"
io8_100m_ft_hs_pd_3v3  "IO8_FT 100MHz high speed @ 3.3V pulldown"
io8_100m_ft_fs_3v3  "IO8_FT 100MHz fast speed @ 3.3V"
io8_100m_ft_fs_pu_3v3  "IO8_FT 100MHz fast speed @ 3.3V pullup"
io8_100m_ft_fs_pd_3v3  "IO8_FT 100MHz fast speed @ 3.3V pulldown"
io8_100m_ft_ms_3v3  "IO8_FT 100MHz med speed @ 3.3V"
io8_100m_ft_ms_pu_3v3  "IO8_FT 100MHz med speed @ 3.3V pullup"
io8_100m_ft_ms_pd_3v3  "IO8_FT 100MHz med speed @ 3.3V pulldown"
io8_100m_ft_ls_3v3  "IO8_FT 100MHz low speed @ 3.3V"
io8_100m_ft_ls_pu_3v3  "IO8_FT 100MHz low speed @ 3.3V pullup"
io8_100m_ft_ls_pd_3v3  "IO8_FT 100MHz low speed @ 3.3V pulldown"
io8usb_adp "IOUSB ADP @ 3.3V"
io8usb_vbus "IOUSB VBUS @ 3.3V"
[Model Selector] io8_usb_ft
io8_100m_ft_hs_1v2  "IO8_FT 100MHz high speed @ 1.2V"
io8_100m_ft_hs_pu_1v2  "IO8_FT 100MHz high speed @ 1.2V pullup"
io8_100m_ft_hs_pd_1v2  "IO8_FT 100MHz high speed @ 1.2V pulldown"
io8_100m_ft_fs_1v2  "IO8_FT 100MHz fast speed @ 1.2V"
io8_100m_ft_fs_pu_1v2  "IO8_FT 100MHz fast speed @ 1.2V pullup"
io8_100m_ft_fs_pd_1v2  "IO8_FT 100MHz fast speed @ 1.2V pulldown"
io8_100m_ft_ms_1v2  "IO8_FT 100MHz med speed @ 1.2V"
io8_100m_ft_ms_pu_1v2  "IO8_FT 100MHz med speed @ 1.2V pullup"
io8_100m_ft_ms_pd_1v2  "IO8_FT 100MHz med speed @ 1.2V pulldown"
io8_100m_ft_ls_1v2  "IO8_FT 100MHz low speed @ 1.2V"
io8_100m_ft_ls_pu_1v2  "IO8_FT 100MHz low speed @ 1.2V pullup"
io8_100m_ft_ls_pd_1v2  "IO8_FT 100MHz low speed @ 1.2V pulldown"
io8_100m_ft_hs_1v8  "IO8_FT 100MHz high speed @ 1.8V"
io8_100m_ft_hs_pu_1v8  "IO8_FT 100MHz high speed @ 1.8V pullup"
io8_100m_ft_hs_pd_1v8  "IO8_FT 100MHz high speed @ 1.8V pulldown"
io8_100m_ft_fs_1v8  "IO8_FT 100MHz fast speed @ 1.8V"
io8_100m_ft_fs_pu_1v8  "IO8_FT 100MHz fast speed @ 1.8V pullup"
io8_100m_ft_fs_pd_1v8  "IO8_FT 100MHz fast speed @ 1.8V pulldown"
io8_100m_ft_ms_1v8  "IO8_FT 100MHz med speed @ 1.8V"
io8_100m_ft_ms_pu_1v8  "IO8_FT 100MHz med speed @ 1.8V pullup"
io8_100m_ft_ms_pd_1v8  "IO8_FT 100MHz med speed @ 1.8V pulldown"
io8_100m_ft_ls_1v8  "IO8_FT 100MHz low speed @ 1.8V"
io8_100m_ft_ls_pu_1v8  "IO8_FT 100MHz low speed @ 1.8V pullup"
io8_100m_ft_ls_pd_1v8  "IO8_FT 100MHz low speed @ 1.8V pulldown"
io8_100m_ft_hs_3v3  "IO8_FT 100MHz high speed @ 3.3V"
io8_100m_ft_hs_pu_3v3  "IO8_FT 100MHz high speed @ 3.3V pullup"
io8_100m_ft_hs_pd_3v3  "IO8_FT 100MHz high speed @ 3.3V pulldown"
io8_100m_ft_fs_3v3  "IO8_FT 100MHz fast speed @ 3.3V"
io8_100m_ft_fs_pu_3v3  "IO8_FT 100MHz fast speed @ 3.3V pullup"
io8_100m_ft_fs_pd_3v3  "IO8_FT 100MHz fast speed @ 3.3V pulldown"
io8_100m_ft_ms_3v3  "IO8_FT 100MHz med speed @ 3.3V"
io8_100m_ft_ms_pu_3v3  "IO8_FT 100MHz med speed @ 3.3V pullup"
io8_100m_ft_ms_pd_3v3  "IO8_FT 100MHz med speed @ 3.3V pulldown"
io8_100m_ft_ls_3v3  "IO8_FT 100MHz low speed @ 3.3V"
io8_100m_ft_ls_pu_3v3  "IO8_FT 100MHz low speed @ 3.3V pullup"
io8_100m_ft_ls_pd_3v3  "IO8_FT 100MHz low speed @ 3.3V pulldown"
io8_usb_fs_3v3  "IOUSB fast speed @ 3.3V"
io8_usb_fs_pu1_3v3  "IO8USB fast speed @ 3.3V pullup1"
io8_usb_fs_pd1_3v3  "IOUSB fast speed @ 3.3V pulldown1"
io8_usb_ls_3v3  "IOUSB low speed @ 3.3V"
io8_usb_ls_pu1_3v3  "IOUSB low speed @ 3.3V pullup1"
io8_usb_ls_pd1_3v3  "IOUSB low speed @ 3.3V pulldown1"
io8_usb_fs_pu2_3v3  "IOUSB fast speed @ 3.3V pullup2"
io8_usb_fs_pd2_3v3  "IOUSB fast speed @ 3.3V pulldown2"
io8_usb_ls_pu2_3v3  "IOUSB low speed @ 3.3V pullup2"
io8_usb_ls_pd2_3v3  "IOUSB low speed @ 3.3V pulldown2"
[Model Selector] io8_100m_i2c_ft
io8_100m_ft_hs_1v2  "IO8_FT 100MHz high speed @ 1.2V"
io8_100m_ft_hs_pu_1v2  "IO8_FT 100MHz high speed @ 1.2V pullup"
io8_100m_ft_hs_pd_1v2  "IO8_FT 100MHz high speed @ 1.2V pulldown"
io8_100m_ft_fs_1v2  "IO8_FT 100MHz fast speed @ 1.2V"
io8_100m_ft_fs_pu_1v2  "IO8_FT 100MHz fast speed @ 1.2V pullup"
io8_100m_ft_fs_pd_1v2  "IO8_FT 100MHz fast speed @ 1.2V pulldown"
io8_100m_ft_ms_1v2  "IO8_FT 100MHz med speed @ 1.2V"
io8_100m_ft_ms_pu_1v2  "IO8_FT 100MHz med speed @ 1.2V pullup"
io8_100m_ft_ms_pd_1v2  "IO8_FT 100MHz med speed @ 1.2V pulldown"
io8_100m_ft_ls_1v2  "IO8_FT 100MHz low speed @ 1.2V"
io8_100m_ft_ls_pu_1v2  "IO8_FT 100MHz low speed @ 1.2V pullup"
io8_100m_ft_ls_pd_1v2  "IO8_FT 100MHz low speed @ 1.2V pulldown"
io8_100m_ft_hs_1v8  "IO8_FT 100MHz high speed @ 1.8V"
io8_100m_ft_hs_pu_1v8  "IO8_FT 100MHz high speed @ 1.8V pullup"
io8_100m_ft_hs_pd_1v8  "IO8_FT 100MHz high speed @ 1.8V pulldown"
io8_100m_ft_fs_1v8  "IO8_FT 100MHz fast speed @ 1.8V"
io8_100m_ft_fs_pu_1v8  "IO8_FT 100MHz fast speed @ 1.8V pullup"
io8_100m_ft_fs_pd_1v8  "IO8_FT 100MHz fast speed @ 1.8V pulldown"
io8_100m_ft_ms_1v8  "IO8_FT 100MHz med speed @ 1.8V"
io8_100m_ft_ms_pu_1v8  "IO8_FT 100MHz med speed @ 1.8V pullup"
io8_100m_ft_ms_pd_1v8  "IO8_FT 100MHz med speed @ 1.8V pulldown"
io8_100m_ft_ls_1v8  "IO8_FT 100MHz low speed @ 1.8V"
io8_100m_ft_ls_pu_1v8  "IO8_FT 100MHz low speed @ 1.8V pullup"
io8_100m_ft_ls_pd_1v8  "IO8_FT 100MHz low speed @ 1.8V pulldown"
io8_100m_ft_hs_3v3  "IO8_FT 100MHz high speed @ 3.3V"
io8_100m_ft_hs_pu_3v3  "IO8_FT 100MHz high speed @ 3.3V pullup"
io8_100m_ft_hs_pd_3v3  "IO8_FT 100MHz high speed @ 3.3V pulldown"
io8_100m_ft_fs_3v3  "IO8_FT 100MHz fast speed @ 3.3V"
io8_100m_ft_fs_pu_3v3  "IO8_FT 100MHz fast speed @ 3.3V pullup"
io8_100m_ft_fs_pd_3v3  "IO8_FT 100MHz fast speed @ 3.3V pulldown"
io8_100m_ft_ms_3v3  "IO8_FT 100MHz med speed @ 3.3V"
io8_100m_ft_ms_pu_3v3  "IO8_FT 100MHz med speed @ 3.3V pullup"
io8_100m_ft_ms_pd_3v3  "IO8_FT 100MHz med speed @ 3.3V pulldown"
io8_100m_ft_ls_3v3  "IO8_FT 100MHz low speed @ 3.3V"
io8_100m_ft_ls_pu_3v3  "IO8_FT 100MHz low speed @ 3.3V pullup"
io8_100m_ft_ls_pd_3v3  "IO8_FT 100MHz low speed @ 3.3V pulldown"
io8_100m_i2c_ft_1v2  "IO8_FT 100MHz I2C @ 1.2V"
io8_100m_i2c_ft_pu_1v2  "IO8_FT 100MHz I2C @ 1.2V pullup"
io8_100m_i2c_ft_pd_1v2  "IO8_FT 100MHz I2C @ 1.2V pulldown"
io8_100m_i2c_ft_1v8  "IO8_FT 100MHz I2C @ 1.8V"
io8_100m_i2c_ft_pu_1v8  "IO8_FT 100MHz I2C @ 1.8V pullup"
io8_100m_i2c_ft_pd_1v8  "IO8_FT 100MHz I2C @ 1,8V pulldown"
io8_100m_i2c_ft_3v3  "IO8_FT 100MHz I2C @ 3.3V"
io8_100m_i2c_ft_pu_3v3  "IO8_FT 100MHz I2C HSLV @ 3.3V pullup"
io8_100m_i2c_ft_pd_3v3  "IO8_FT 100MHz I2C @ 3.3V pulldown"
[Model Selector] io8_166m_hslv_i2c_ft
io8_166m_ft_hs_1v2  "IO8_FT 166MHz high speed @ 1.2V"
io8_166m_ft_hs_pu_1v2  "IO8_FT 166MHz high speed @ 1.2V pullup"
io8_166m_ft_hs_pd_1v2  "IO8_FT 166MHz high speed @ 1.2V pulldown"
io8_166m_ft_fs_1v2  "IO8_FT 166MHz fast speed @ 1.2V"
io8_166m_ft_fs_pu_1v2  "IO8_FT 166MHz fast speed @ 1.2V pullup"
io8_166m_ft_fs_pd_1v2  "IO8_FT 166MHz fast speed @ 1.2V pulldown"
io8_166m_ft_ms_1v2  "IO8_FT 166MHz med speed @ 1.2V"
io8_166m_ft_ms_pu_1v2  "IO8_FT 166MHz med speed @ 1.2V pullup"
io8_166m_ft_ms_pd_1v2  "IO8_FT 166MHz med speed @ 1.2V pulldown"
io8_166m_ft_ls_1v2  "IO8_FT 166MHz low speed @ 1.2V"
io8_166m_ft_ls_pu_1v2  "IO8_FT 166MHz low speed @ 1.2V pullup"
io8_166m_ft_ls_pd_1v2  "IO8_FT 166MHz low speed @ 1.2V pulldown"
io8_166m_ft_hs_1v8  "IO8_FT 166MHz high speed @ 1.8V"
io8_166m_ft_hs_pu_1v8  "IO8_FT 166MHz high speed @ 1.8V pullup"
io8_166m_ft_hs_pd_1v8  "IO8_FT 166MHz high speed @ 1.8V pulldown"
io8_166m_ft_fs_1v8  "IO8_FT 166MHz fast speed @ 1.8V"
io8_166m_ft_fs_pu_1v8  "IO8_FT 166MHz fast speed @ 1.8V pullup"
io8_166m_ft_fs_pd_1v8  "IO8_FT 166MHz fast speed @ 1.8V pulldown"
io8_166m_ft_ms_1v8  "IO8_FT 166MHz med speed @ 1.8V"
io8_166m_ft_ms_pu_1v8  "IO8_FT 166MHz med speed @ 1.8V pullup"
io8_166m_ft_ms_pd_1v8  "IO8_FT 166MHz med speed @ 1.8V pulldown"
io8_166m_ft_ls_1v8  "IO8_FT 166MHz low speed @ 1.8V"
io8_166m_ft_ls_pu_1v8  "IO8_FT 166MHz low speed @ 1.8V pullup"
io8_166m_ft_ls_pd_1v8  "IO8_FT 166MHz low speed @ 1.8V pulldown"
io8_166m_ft_hs_3v3  "IO8_FT 166MHz high speed @ 3.3V"
io8_166m_ft_hs_pu_3v3  "IO8_FT 166MHz high speed @ 3.3V pullup"
io8_166m_ft_hs_pd_3v3  "IO8_FT 166MHz high speed @ 3.3V pulldown"
io8_166m_ft_fs_3v3  "IO8_FT 166MHz fast speed @ 3.3V"
io8_166m_ft_fs_pu_3v3  "IO8_FT 166MHz fast speed @ 3.3V pullup"
io8_166m_ft_fs_pd_3v3  "IO8_FT 166MHz fast speed @ 3.3V pulldown"
io8_166m_ft_ms_3v3  "IO8_FT 166MHz med speed @ 3.3V"
io8_166m_ft_ms_pu_3v3  "IO8_FT 166MHz med speed @ 3.3V pullup"
io8_166m_ft_ms_pd_3v3  "IO8_FT 166MHz med speed @ 3.3V pulldown"
io8_166m_ft_ls_3v3  "IO8_FT 166MHz low speed @ 3.3V"
io8_166m_ft_ls_pu_3v3  "IO8_FT 166MHz low speed @ 3.3V pullup"
io8_166m_ft_ls_pd_3v3  "IO8_FT 166MHz low speed @ 3.3V pulldown"
io8_166m_hslv_ft_hs_1v2  "IO8_FT 166MHz HSLV high speed @ 1.2V"
io8_166m_hslv_ft_hs_pu_1v2  "IO8_FT 166MHz HSLV high speed @ 1.2V pullup"
io8_166m_hslv_ft_hs_pd_1v2  "IO8_FT 166MHz HSLV high speed @ 1.2V pulldown"
io8_166m_hslv_ft_fs_1v2  "IO8_FT 166MHz HSLV fast speed @ 1.2V"
io8_166m_hslv_ft_fs_pu_1v2  "IO8_FT 166MHz HSLV fast speed @ 1.2V pullup"
io8_166m_hslv_ft_fs_pd_1v2  "IO8_FT 166MHz HSLV fast speed @ 1.2V pulldown"
io8_166m_hslv_ft_ms_1v2  "IO8_FT 166MHz HSLV med speed @ 1.2V"
io8_166m_hslv_ft_ms_pu_1v2  "IO8_FT 166MHz HSLV med speed @ 1.2V pullup"
io8_166m_hslv_ft_ms_pd_1v2  "IO8_FT 166MHz HSLV med speed @ 1.2V pulldown"
io8_166m_hslv_ft_ls_1v2  "IO8_FT 166MHz HSLV low speed @ 1.2V"
io8_166m_hslv_ft_ls_pu_1v2  "IO8_FT 166MHz HSLV low speed @ 1.2V pullup"
io8_166m_hslv_ft_ls_pd_1v2  "IO8_FT 166MHz HSLV low speed @ 1.2V pulldown"
io8_166m_hslv_ft_hs_1v8  "IO8_FT 166MHz HSLV high speed @ 1.8V"
io8_166m_hslv_ft_hs_pu_1v8  "IO8_FT 166MHz HSLV high speed @ 1.8V pullup"
io8_166m_hslv_ft_hs_pd_1v8  "IO8_FT 166MHz HSLV high speed @ 1.8V pulldown"
io8_166m_hslv_ft_fs_1v8  "IO8_FT 166MHz HSLV fast speed @ 1.8V"
io8_166m_hslv_ft_fs_pu_1v8  "IO8_FT 166MHz HSLV fast speed @ 1.8V pullup"
io8_166m_hslv_ft_fs_pd_1v8  "IO8_FT 166MHz HSLV fast speed @ 1.8V pulldown"
io8_166m_hslv_ft_ms_1v8  "IO8_FT 166MHz HSLV med speed @ 1.8V"
io8_166m_hslv_ft_ms_pu_1v8  "IO8_FT 166MHz HSLV med speed @ 1.8V pullup"
io8_166m_hslv_ft_ms_pd_1v8  "IO8_FT 166MHz HSLV med speed @ 1.8V pulldown"
io8_166m_hslv_ft_ls_1v8  "IO8_FT 166MHz HSLV low speed @ 1.8V"
io8_166m_hslv_ft_ls_pu_1v8  "IO8_FT 166MHz HSLV low speed @ 1.8V pullup"
io8_166m_hslv_ft_ls_pd_1v8  "IO8_FT 166MHz HSLV low speed @ 1.8V pulldown"
io8_166m_hslv_ft_hs_2v5  "IO8_FT 166MHz HSLV high speed @ 2.5V"
io8_166m_hslv_ft_hs_pu_2v5  "IO8_FT 166MHz HSLV high speed @ 2.5V pullup"
io8_166m_hslv_ft_hs_pd_2v5  "IO8_FT 166MHz HSLV high speed @ 2.5V pulldown"
io8_166m_hslv_ft_fs_2v5  "IO8_FT 166MHz HSLV fast speed @ 2.5V"
io8_166m_hslv_ft_fs_pu_2v5  "IO8_FT 166MHz HSLV fast speed @ 2.5V pullup"
io8_166m_hslv_ft_fs_pd_2v5  "IO8_FT 166MHz HSLV fast speed @ 2.5V pulldown"
io8_166m_hslv_ft_ms_2v5  "IO8_FT 166MHz HSLV med speed @ 2.5V"
io8_166m_hslv_ft_ms_pu_2v5  "IO8_FT 166MHz HSLV med speed @ 2.5V pullup"
io8_166m_hslv_ft_ms_pd_2v5  "IO8_FT 166MHz HSLV med speed @ 2.5V pulldown"
io8_166m_hslv_ft_ls_2v5  "IO8_FT 166MHz HSLV low speed @ 2.5V"
io8_166m_hslv_ft_ls_pu_2v5  "IO8_FT 166MHz HSLV low speed @ 2.5V pullup"
io8_166m_hslv_ft_ls_pd_2v5  "IO8_FT 166MHz HSLV low speed @ 2.5V pulldown"
io8_166m_i2c_ft_1v2  "IO8_FT 166MHz I2C @ 1.2V"
io8_166m_i2c_ft_pu_1v2  "IO8_FT 166MHz I2C @ 1.2V pullup"
io8_166m_i2c_ft_pd_1v2  "IO8_FT 166MHz I2C @ 1.2V pulldown"
io8_166m_i2c_ft_1v8  "IO8_FT 166MHz I2C @ 1.8V"
io8_166m_i2c_ft_pu_1v8  "IO8_FT 166MHz I2C @ 1.8V pullup"
io8_166m_i2c_ft_pd_1v8  "IO8_FT 166MHz I2C @ 1,8V pulldown"
io8_166m_i2c_ft_3v3  "IO8_FT 166MHz I2C @ 3.3V"
io8_166m_i2c_ft_pu_3v3  "IO8_FT 166MHz I2C HSLV @ 3.3V pullup"
io8_166m_i2c_ft_pd_3v3  "IO8_FT 166MHz I2C @ 3.3V pulldown"
| Models and submodels in the file (212): io8_100m_ft_hs_1v2 (I/O), io8_100m_ft_hs_pu_1v2 (I/O), io8_100m_ft_hs_pd_1v2 (I/O), io8_100m_ft_fs_1v2 (I/O), io8_100m_ft_fs_pu_1v2 (I/O), io8_100m_ft_fs_pd_1v2 (I/O), io8_100m_ft_ms_1v2 (I/O), io8_100m_ft_ms_pu_1v2 (I/O), io8_100m_ft_ms_pd_1v2 (I/O), io8_100m_ft_ls_1v2 (I/O), io8_100m_ft_ls_pu_1v2 (I/O), io8_100m_ft_ls_pd_1v2 (I/O), io8_100m_ft_hs_1v8 (I/O), io8_100m_ft_hs_pu_1v8 (I/O), io8_100m_ft_hs_pd_1v8 (I/O), io8_100m_ft_fs_1v8 (I/O), io8_100m_ft_fs_pu_1v8 (I/O), io8_100m_ft_fs_pd_1v8 (I/O), io8_100m_ft_ms_1v8 (I/O), io8_100m_ft_ms_pu_1v8 (I/O), io8_100m_ft_ms_pd_1v8 (I/O), io8_100m_ft_ls_1v8 (I/O), io8_100m_ft_ls_pu_1v8 (I/O), io8_100m_ft_ls_pd_1v8 (I/O), io8_100m_ft_hs_3v3 (I/O), io8_100m_ft_hs_pu_3v3 (I/O), io8_100m_ft_hs_pd_3v3 (I/O), io8_100m_ft_fs_3v3 (I/O), io8_100m_ft_fs_pu_3v3 (I/O), io8_100m_ft_fs_pd_3v3 (I/O), io8_100m_ft_ms_3v3 (I/O), io8_100m_ft_ms_pu_3v3 (I/O), io8_100m_ft_ms_pd_3v3 (I/O), io8_100m_ft_ls_3v3 (I/O), io8_100m_ft_ls_pu_3v3 (I/O), io8_100m_ft_ls_pd_3v3 (I/O), io8_100m_hslv_ft_hs_1v2 (I/O), io8_100m_hslv_ft_hs_pu_1v2 (I/O), io8_100m_hslv_ft_hs_pd_1v2 (I/O), io8_100m_hslv_ft_fs_1v2 (I/O), io8_100m_hslv_ft_fs_pu_1v2 (I/O), io8_100m_hslv_ft_fs_pd_1v2 (I/O), io8_100m_hslv_ft_ms_1v2 (I/O), io8_100m_hslv_ft_ms_pu_1v2 (I/O), io8_100m_hslv_ft_ms_pd_1v2 (I/O), io8_100m_hslv_ft_ls_1v2 (I/O), io8_100m_hslv_ft_ls_pu_1v2 (I/O), io8_100m_hslv_ft_ls_pd_1v2 (I/O), io8_100m_hslv_ft_hs_1v8 (I/O), io8_100m_hslv_ft_hs_pu_1v8 (I/O), io8_100m_hslv_ft_hs_pd_1v8 (I/O), io8_100m_hslv_ft_fs_1v8 (I/O), io8_100m_hslv_ft_fs_pu_1v8 (I/O), io8_100m_hslv_ft_fs_pd_1v8 (I/O), io8_100m_hslv_ft_ms_1v8 (I/O), io8_100m_hslv_ft_ms_pu_1v8 (I/O), io8_100m_hslv_ft_ms_pd_1v8 (I/O), io8_100m_hslv_ft_ls_1v8 (I/O), io8_100m_hslv_ft_ls_pu_1v8 (I/O), io8_100m_hslv_ft_ls_pd_1v8 (I/O), io8_100m_hslv_ft_hs_2v5 (I/O), io8_100m_hslv_ft_hs_pu_2v5 (I/O), io8_100m_hslv_ft_hs_pd_2v5 (I/O), io8_100m_hslv_ft_fs_2v5 (I/O), io8_100m_hslv_ft_fs_pu_2v5 (I/O), io8_100m_hslv_ft_fs_pd_2v5 (I/O), io8_100m_hslv_ft_ms_2v5 (I/O), io8_100m_hslv_ft_ms_pu_2v5 (I/O), io8_100m_hslv_ft_ms_pd_2v5 (I/O), io8_100m_hslv_ft_ls_2v5 (I/O), io8_100m_hslv_ft_ls_pu_2v5 (I/O), io8_100m_hslv_ft_ls_pd_2v5 (I/O), io8_166m_ft_hs_1v2 (I/O), io8_166m_ft_hs_pu_1v2 (I/O), io8_166m_ft_hs_pd_1v2 (I/O), io8_166m_ft_fs_1v2 (I/O), io8_166m_ft_fs_pu_1v2 (I/O), io8_166m_ft_fs_pd_1v2 (I/O), io8_166m_ft_ms_1v2 (I/O), io8_166m_ft_ms_pu_1v2 (I/O)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
